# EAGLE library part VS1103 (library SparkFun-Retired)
MIDI/ADPCM/WAV codec, MIDI synth Retired -- Stock still available but looks EOL
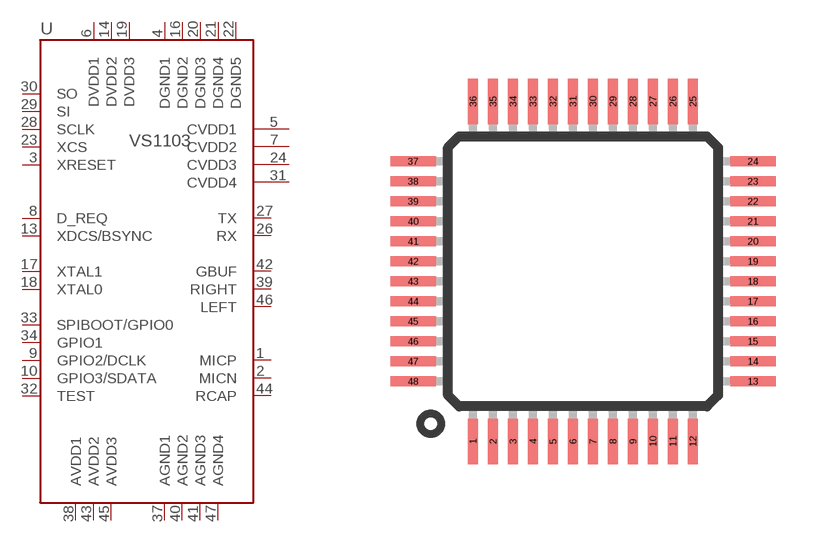
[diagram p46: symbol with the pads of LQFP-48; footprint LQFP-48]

Designator prefix -

## VS1103  [LQFP-48]
1  MICP
2  MICN
3  XRESET
4  DGND1  pwr
5  CVDD1
6  DVDD1  pwr
7  CVDD2
8  D_REQ
9  GPIO2/DCLK
10  GPIO3/SDATA
13  XDCS/BSYNC
14  DVDD2  pwr
16  DGND2
17  XTAL1
18  XTAL0
19  DVDD3  pwr
20  DGND3
21  DGND4
22  DGND5
23  XCS
24  CVDD3
26  RX
27  TX
28  SCLK
29  SI
30  SO
31  CVDD4
32  TEST
33  SPIBOOT/GPIO0
34  GPIO1
37  AGND1
38  AVDD1  pwr
39  RIGHT
40  AGND2
41  AGND3
42  GBUF
43  AVDD2  pwr
44  RCAP
45  AVDD3  pwr
46  LEFT
47  AGND4

## Footprint LQFP-48 (pad centres in mm)
smd 0.254 x 1.143: 1 -2.75,-4.25; 2 -2.25,-4.25; 3 -1.75,-4.25; 4 -1.25,-4.25; 5 -0.75,-4.25; 6 -0.25,-4.25; 7 0.25,-4.25; 8 0.75,-4.25; 9 1.25,-4.25; 10 1.75,-4.25; 11 2.25,-4.25; 12 2.75,-4.25; 25 2.75,4.25; 26 2.25,4.25; 27 1.75,4.25; 28 1.25,4.25; 29 0.75,4.25; 30 0.25,4.25; 31 -0.25,4.25; 32 -0.75,4.25; 33 -1.25,4.25; 34 -1.75,4.25; 35 -2.25,4.25; 36 -2.75,4.25
smd 1.143 x 0.254: 13 4.25,-2.75; 14 4.25,-2.25; 15 4.25,-1.75; 16 4.25,-1.25; 17 4.25,-0.75; 18 4.25,-0.25; 19 4.25,0.25; 20 4.25,0.75; 21 4.25,1.25; 22 4.25,1.75; 23 4.25,2.25; 24 4.25,2.75; 37 -4.25,2.75; 38 -4.25,2.25; 39 -4.25,1.75; 40 -4.25,1.25; 41 -4.25,0.75; 42 -4.25,0.25; 43 -4.25,-0.25; 44 -4.25,-0.75; 45 -4.25,-1.25; 46 -4.25,-1.75; 47 -4.25,-2.25; 48 -4.25,-2.75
